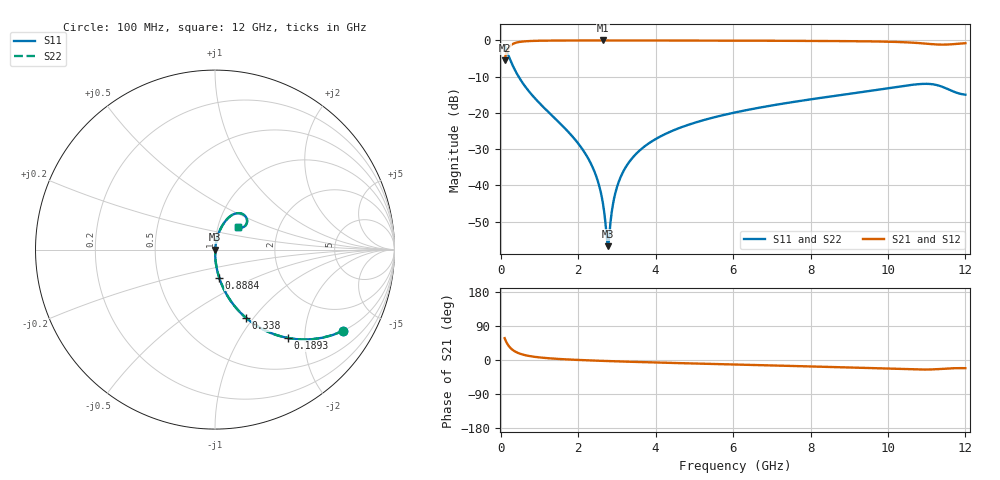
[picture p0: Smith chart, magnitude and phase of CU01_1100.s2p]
! S-parameter model data by Modelithics Inc. support@modelithics.com 813-866-6335 Tampa FL USA
! S-Parameter data specifications:
! Substrate: 20-mil Rogers, substrate thickness, H=0.508mm, Dielectric constant, Er=3.75
! PCB Mounting Pad Footprint: Pad width, PadW=0.35mm , Pad length, PadL=0.30mm , Pad gap, PadG (edge-to-edge)=0.25mm , Reference planes=0.85mm apart
! Created Tue May  8 14:01:25 2018
# hz S ma R 50
! 2 Port Network Data from SP1.SP block
! freq  magS11  angS11  magS21  angS21  magS12  angS12  magS22  angS22
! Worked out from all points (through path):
!   801 points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, 100 MHz to 12 GHz, reference 50 ohm
!   highest |S21| = -0.01 dB at 2.629 GHz (marker M1); lowest = -5.4 dB at 100 MHz (marker M2)
!   group delay of S21, straight-line fit = 9.07 ps
!   lowest |S11| = -56.8 dB at 2.763 GHz (marker M3), VSWR 1.00, Z = 50.1 - j0.0291 ohm
!   |S11| at or under -10 dB: 462 MHz to end of sweep
!   |S22| runs from -56.8 to -1.5 dB; largest |S21 - S12| = 0
!   S11 on the Smith chart (normalised r, x): 100 MHz: 1.00, -3.16; 189.2 MHz: 1.00, -1.66; 338 MHz: 1.00, -0.92; 888.4 MHz: 1.00, -0.32; 12 GHz: 1.24, +0.32
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1e8  0.8452 -32.4  0.534 57.6  0.534 57.6  0.8452 -32.4
1.8925e8  0.64 -50.4  0.7679 39.6  0.7679 39.6  0.64 -50.4
3.38e8  0.4191 -65.5  0.9074 24.4  0.9074 24.4  0.4191 -65.5
5.31375e8  0.2759 -74.4  0.9605 15.5  0.9605 15.5  0.2759 -74.4
8.88375e8  0.158 -81.5  0.9866 8.2  0.9866 8.2  0.158 -81.5
2.09325e9  0.03248 -88.0  0.9982 -0.3  0.9982 -0.3  0.03248 -88.0
2.435375e9  0.0148 -86.4  0.9985 -1.6  0.9985 -1.6  0.0148 -86.4
2.5395e9  0.01001 -84.1  0.9985 -2.0  0.9985 -2.0  0.01001 -84.1
2.62875e9  0.006096 -79.0  0.9985 -2.3  0.9985 -2.3  0.006096 -79.0
2.718e9  0.002532 -58.4  0.9985 -2.6  0.9985 -2.6  0.002532 -58.4
2.762625e9  0.001452 -11.5  0.9985 -2.8  0.9985 -2.8  0.001452 -11.5
2.80725e9  0.002174 45.4  0.9985 -3.0  0.9985 -3.0  0.002174 45.4
2.881625e9  0.00486 69.3  0.9985 -3.2  0.9985 -3.2  0.00486 69.3
2.956e9  0.007716 75.5  0.9984 -3.4  0.9984 -3.4  0.007716 75.5
3.16425e9  0.01554 80.2  0.9983 -4.1  0.9983 -4.1  0.01554 80.2
3.52125e9  0.02809 81.5  0.9979 -5.2  0.9979 -5.2  0.02809 81.5
4.071625e9  0.0458 81.1  0.9972 -6.8  0.9972 -6.8  0.0458 81.1
6.05e9  0.1014 76.7  0.9925 -12.0  0.9925 -12.0  0.1014 76.7
8.04325e9  0.1549 71.5  0.984 -17.1  0.984 -17.1  0.1549 71.5
1.002162e10  0.2194 62.9  0.9593 -22.8  0.9593 -22.8  0.2194 62.9
1.109262e10  0.2504 46.5  0.8919 -25.0  0.8919 -25.0  0.2504 46.5
1.2e10  0.1784 44.8  0.915 -21.6  0.915 -21.6  0.1784 44.8
